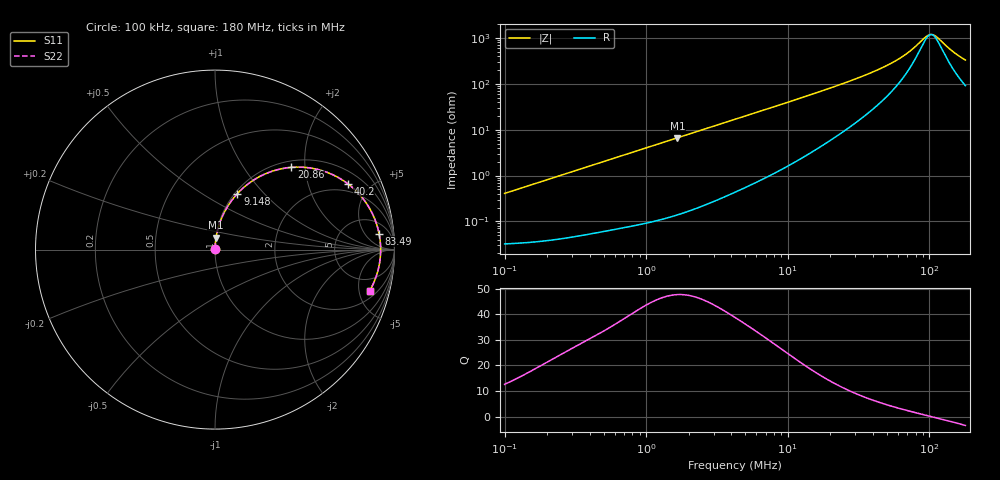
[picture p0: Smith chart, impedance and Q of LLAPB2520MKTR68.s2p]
! LLAPB2520MKTR68  S-PARAMETER MODEL  ( General Type )
! Model Generated by TAIYO YUDEN Corporation (http://www.ty-top.com)
! Version 1.0
! TAIYO YUDEN Control No. 151211NG33SB-FKC
! Copyright(c) 2015 TAIYO YUDEN CO.,LTD. All Rights Reserved.
! Product Description (link to TY-COMPAS)
! https://ds.yuden.co.jp/TYCOMPAS/or/detail?pn=LLAPB2520MKTR68M&u=M
! Products Name : Inductors
! Characteristics :
!  Inductance : 0.68 uH , SRF(min) : -Hz , DC Resistance(max) : 0.036 Ohm
!  Rated Current : Saturation :5100 mA , Temp Rise : 3500 mA (40 degC)
!  Case Size : 2.5 x 2.0 / 0.098 x 0.079 [mm/inch] , Thickness : 1.2 / 0.047 [mm/inch]
!  (Conditions: Temperature = 25 degC , DC Bias Current/Voltage = 0A / 0V)
! External Node Assignments :
!  1  o---GGG---o  2
! GND o---------o GND
! Frequency Range : 0.1MHz  -  180.004543MHz  [ 402 STEP ]
# MHz S RI R 50
! Freq[MHz].  S11 Real  S11 Imag  S21 Real  S21 Imag  S12 Real  S12 Imag  S22 Real  S22 Imag
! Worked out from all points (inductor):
!   401 points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, 100 kHz to 180 MHz, reference 50 ohm
!   read as one part in series: L = 647 nH near 103.8 kHz
!   highest Q = 47.7 at 1.662 MHz (marker M1), where L = 633 nH
!   self-resonance near 103.1 MHz
!   S11 on the Smith chart (normalised r, x): 100 kHz: 1.00, +0.01; 9.148 MHz: 1.03, +0.72; 20.86 MHz: 1.13, +1.70; 40.2 MHz: 1.57, +3.62; 83.49 MHz: 10, +12; 180 MHz: 2.83, -6.37
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0.1  0.000339 0.00406  0.9997 -0.00406  0.9997 -0.00406  0.000339 0.00406
0.350962  0.000693 0.0141  0.9993 -0.0141  0.9993 -0.0141  0.000693 0.0141
1.231743  0.00346 0.0488  0.9965 -0.0488  0.9965 -0.0488  0.00346 0.0488
1.662384  0.00571 0.0656  0.9943 -0.0656  0.9943 -0.0656  0.00571 0.0656
2.757166  0.0142 0.1075  0.9858 -0.1075  0.9858 -0.1075  0.0142 0.1075
4.322947  0.0324 0.1646  0.9676 -0.1646  0.9676 -0.1646  0.0324 0.1646
6.528607  0.0689 0.2381  0.9311 -0.2381  0.9311 -0.2381  0.0689 0.2381
9.147624  0.125 0.3122  0.875 -0.3122  0.875 -0.3122  0.125 0.3122
11.67092  0.1876 0.3684  0.8124 -0.3684  0.8124 -0.3684  0.1876 0.3684
14.89024  0.2728 0.4187  0.7272 -0.4187  0.7272 -0.4187  0.2728 0.4187
20.86361  0.4251 0.4582  0.5749 -0.4582  0.5749 -0.4582  0.4251 0.4582
28.69056  0.5861 0.443  0.4139 -0.443  0.4139 -0.443  0.5861 0.443
40.20007  0.7397 0.3672  0.2603 -0.3672  0.2603 -0.3672  0.7397 0.3672
52.25907  0.8294 0.2778  0.1706 -0.2778  0.1706 -0.2778  0.8294 0.2778
67.93547  0.8885 0.1744  0.1115 -0.1744  0.1115 -0.1744  0.8885 0.1744
83.48663  0.9142 0.0889  0.0858 -0.0889  0.0858 -0.0889  0.9142 0.0889
96.98902  0.9222 0.0259  0.0778 -0.0259  0.0778 -0.0259  0.9222 0.0259
102.5976  0.9229 0.00219  0.0771 -0.00219  0.0771 -0.00219  0.9229 0.00219
106.5157  0.9227 -0.0136  0.0773 0.0136  0.0773 0.0136  0.9227 -0.0136
114.8065  0.9207 -0.0452  0.0793 0.0452  0.0793 0.0452  0.9207 -0.0452
149.2455  0.8962 -0.1548  0.1038 0.1548  0.1038 0.1548  0.8962 -0.1548
180.0045  0.8612 -0.2307  0.1388 0.2307  0.1388 0.2307  0.8612 -0.2307
